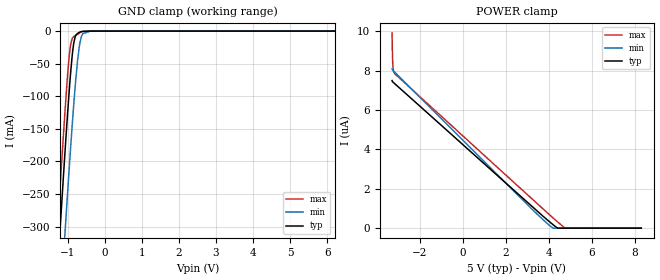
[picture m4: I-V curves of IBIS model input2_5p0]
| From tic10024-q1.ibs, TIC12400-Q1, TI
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|   input2_5p0 Model
[Model]   input2_5p0
Model_type   Input
Vinl = 1.5
Vinh = 3.5
|   typ   min   max
C_comp   1.3729E-12F   1.2991E-12F   1.41789E-12F
[Model spec]
|subparameter
Vinl   1.5   1.35   1.65
Vinh   3.5   3.15   3.85
| Where nom  PVT is Nominal Process, 5.0V, 27C
|   Fast PVT is Strong Process,  5.5V, -40C
|   Slow PVT is Weak Process,   4.5V, 150C
[Voltage Range]   5   4.5   5.5
|Junction Temperature
[Temperature Range]   27   150   -40
[Power Clamp Reference]   5   4.5   5.5
[GND Clamp Reference]   0   0   0
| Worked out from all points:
|   GND clamp passes 1 mA (typ) near -0.65 V on its own axis
[GND Clamp]
|   Voltage   I(typ)   I(min)   I(max)
-3.3V     -2.326A    -2.432A    -2.273A
-1.514V   -590mA     -713.8mA   -527mA
-1.235V   -327.8mA   -452.9mA   -263.8mA
-1.212V   -306.4mA   -431.6mA   -242.5mA
-1.084V   -191.9mA   -316mA     -129.2mA
-1.038V   -152mA     -275mA     -91.03mA
-945.2mV  -78.23mA   -195.5mA   -29.19mA
-840.8mV  -18.6mA    -112.5mA   -8.361mA
-690mV    -1.941mA   -23.55mA   -3.155mA
-597.2mV  -361.4uA   -3.918mA   -593.3uA
-388.4mV  -541.8nA   -27.14uA   -345.9nA
8.3V      0A         0A         0A
[POWER Clamp]
|   Voltage   I(typ)   I(min)   I(max)
-3.3V     7.491uA    8.09uA     9.911uA
-3.288V   7.441uA    8.037uA    9.042uA
-3.277V   7.43uA     8.024uA    8.557uA
-3.265V   7.418uA    8.011uA    8.275uA
-3.242V   7.396uA    7.986uA    8.012uA
-3.184V   7.339uA    7.923uA    7.849uA
3.672V    658.8nA    487.2nA    1.033uA
4.194V    175.9nA    4.64nA     518.1nA
4.402V    5.634nA    0A         318.5nA
4.681V    0A         0A         64.7nA
4.774V    0A         0A         0A
8.3V      0A         0A         0A
